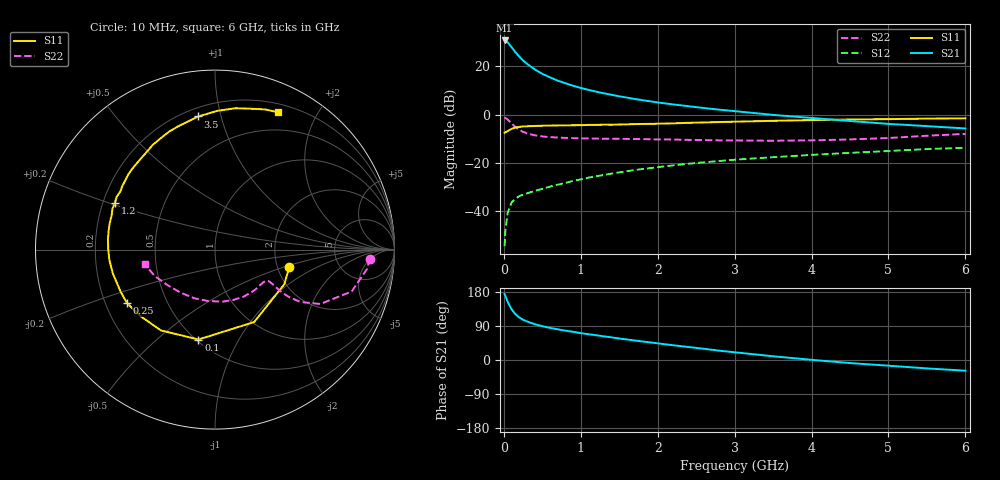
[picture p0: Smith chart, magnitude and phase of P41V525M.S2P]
! SIEMENS Small Signal Semiconductors
! BFP182
! Si NPN RF Bipolar Junction Transistor in SOT143
! VCE = 1.5 V  IC = 25 mA
! Common Emitter S-Parameters:  March  1996
# GHz  S  MA  R  50
!  f  S11  S21  S12  S22
! GHz  MAG  ANG  MAG  ANG  MAG  ANG  MAG  ANG
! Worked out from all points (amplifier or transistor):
!   36 points, 10 MHz to 6 GHz, reference 50 ohm
!   highest |S21| = 30.7 dB at 10 MHz (marker M1)
!   |S21| within 3 dB of that: start of sweep to 105 MHz
!   unconditionally stable (mu >= 1): start of sweep to 16.42 MHz; 322.8 MHz to end of sweep
!   at 250 MHz: K = 0.84, MSG = 27.8 dB, |S12| = -33.1 dB
!   at 1.4 GHz: K = 1.66, MAG = 11.6 dB, |S12| = -24.4 dB
!   at 6 GHz: K = 1.20, MAG = 1.3 dB, |S12| = -13.7 dB
!   S11 on the Smith chart (normalised r, x): 10 MHz: 2.32, -0.56; 100 MHz: 0.51, -0.69; 250 MHz: 0.29, -0.26; 1.2 GHz: 0.25, +0.21; 3.5 GHz: 0.25, +0.85; 6 GHz: 0.29, +1.52
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0.01  0.4254 -13.5  34.43 174.3  0.0019 78.5  0.8638 -3.3
0.02  0.4316 -26.6  34.27 169.1  0.004 73.3  0.8549 -7.1
0.05  0.4588 -61.6  31.56 153.2  0.0094 71.1  0.7968 -17.0
0.1  0.5093 -100.4  24.95 133.8  0.0152 53.9  0.6606 -27.3
0.15  0.5419 -123.8  19.78 121.1  0.0184 48.4  0.5589 -31.5
0.2  0.558 -138.8  15.99 112.4  0.0206 45.5  0.488 -32.7
0.25  0.5738 -148.8  13.27 106.2  0.0221 45.4  0.4416 -32.6
0.3  0.5757 -155.8  11.35 101.8  0.0235 45.0  0.4117 -32.0
0.4  0.5846 -166.7  8.71 94.5  0.0264 47.7  0.3752 -31.0
0.5  0.5913 -174.4  7.004 89.2  0.0292 48.4  0.3547 -30.5
0.6  0.595 179.6  5.938 84.8  0.0325 50.6  0.3434 -30.5
0.7  0.5993 174.5  5.074 81.0  0.0356 52.6  0.3364 -31.2
0.9  0.6051 165.9  3.984 74.4  0.0426 54.5  0.3275 -33.1
1.1  0.6151 158.3  3.269 68.0  0.0499 55.5  0.3223 -36.2
1.2  0.6154 154.8  3 65.4  0.0531 55.2  0.3199 -37.9
1.7  0.6393 139.0  2.113 51.5  0.0716 54.5  0.3135 -47.5
2.2  0.6617 125.8  1.633 38.9  0.0894 51.0  0.3065 -59.2
2.8  0.7056 111.1  1.272 24.6  0.11 46.0  0.2942 -75.4
3.5  0.7475 97.2  0.991 9.8  0.1319 39.5  0.2894 -96.9
4.5  0.7961 81.7  0.741 -8.1  0.1623 30.4  0.3076 -129.0
5.5  0.8296 70.3  0.58 -22.2  0.1945 21.2  0.3669 -156.3
6  0.8417 65.3  0.519 -28.2  0.2066 15.7  0.4006 -168.6
